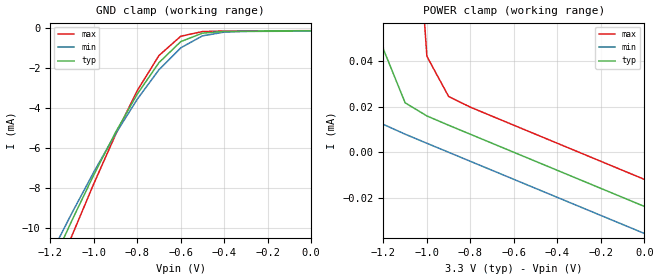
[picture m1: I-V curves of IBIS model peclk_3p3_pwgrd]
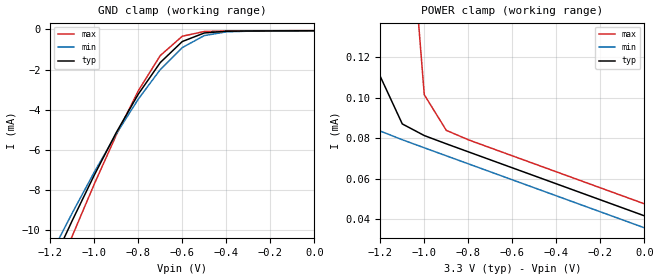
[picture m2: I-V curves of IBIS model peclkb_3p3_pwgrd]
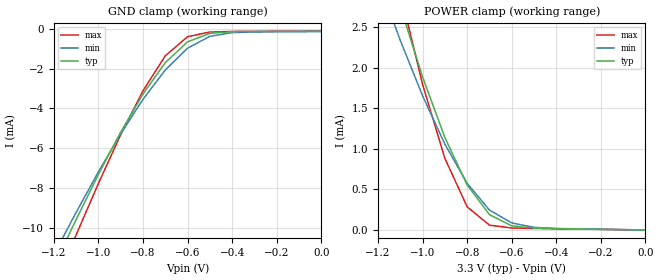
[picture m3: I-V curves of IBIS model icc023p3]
[IBIS ver]   2.1
[File name]   mpc9658.ibs
[File Rev]   2.2 {April 29, 2002}
[Date]   January 9th, 2002
[Disclaimer]   This information is for modeling purposes only
|   and is not guaranteed.
[Source]   Timing Solutions Operations
[Copyright]   Copyright 2001, Motorola Incorporated,
|   all rights reserved.
| Component MPC9658 for 3.3V Application!
[Component]   MPC96583p3
[Manufacturer]   Motorola
[Package]
|   typ   min   max
R_pkg   0.048   .038   0.053
L_pkg   6.045nH   5.084nH   7.950nH
C_pkg   0.813pF   0.560pF   1.157pF
[Pin]   signal_name model_name R_pin L_pin   C_pin
2   FB_IN   icc023p3   0.04   0.35nH   0.053pF
3   BYPASS_BAR  icc023p3   0.04   0.35nH   0.053pF
4   PLL_EN   icc023p3   0.04   0.35nH   0.053pF
5   MR/OEB   icc043p3   0.04   0.35nH   0.053pF
6   PCLK   peclk_3p3_pwgrd   0.04   0.35nH   0.053pF
7   PCLK_BAR   peclkb_3p3_pwgrd   0.04   0.35nH   0.053pF
10   Q9   occ013p3   0.04   0.35nH   0.053pF
12   Q8   occ013p3   0.04   0.35nH   0.053pF
14   Q7   occ013p3   0.04   0.35nH   0.053pF
16   Q6   occ013p3   0.04   0.35nH   0.053pF
18   Q5   occ013p3   0.04   0.35nH   0.053pF
20   Q4   occ013p3   0.04   0.35nH   0.053pF
22   Q3   occ013p3   0.04   0.35nH   0.053pF
24   Q2   occ013p3   0.04   0.35nH   0.053pF
26   Q1   occ013p3   0.04   0.35nH   0.053pF
28   Q0   occ013p3   0.04   0.35nH   0.053pF
30   QA1   occ013p3   0.04   0.35nH   0.053pF
32   VCO_SEL   icc023p3   0.04   0.35nH   0.053pF
|Component Inputs and Outputs at 2.5V Application
[Component]   MPC96582p5
[Manufacturer]   Motorola
[Package]
|   typ   min   max
R_pkg   0.048   .038   0.053
L_pkg   6.045nH   5.084nH   7.950nH
C_pkg   0.813pF   0.560pF   1.157pF
[Pin]   signal_name model_name R_pin L_pin   C_pin
2   FB_IN   icc022p5   0.04   0.35nH   0.053pF
3   BYPASS_BAR  icc022p5   0.04   0.35nH   0.053pF
4   PLL_EN   icc022p5   0.04   0.35nH   0.053pF
5   MR/OEB   icc042p5   0.04   0.35nH   0.053pF
6   PCLK   peclk_2p5_pwgrd   0.04   0.35nH   0.053pF
7   PCLK_BAR   peclkb_2p5_pwgrd   0.04   0.35nH   0.053pF
10   Q9   occ012p5   0.04   0.35nH   0.053pF
12   Q8   occ012p5   0.04   0.35nH   0.053pF
14   Q7   occ012p5   0.04   0.35nH   0.053pF
16   Q6   occ012p5   0.04   0.35nH   0.053pF
18   Q5   occ012p5   0.04   0.35nH   0.053pF
20   Q4   occ012p5   0.04   0.35nH   0.053pF
22   Q3   occ012p5   0.04   0.35nH   0.053pF
24   Q2   occ012p5   0.04   0.35nH   0.053pF
26   Q1   occ012p5   0.04   0.35nH   0.053pF
28   Q0   occ012p5   0.04   0.35nH   0.053pF
30   QA1   occ012p5   0.04   0.35nH   0.053pF
32   VCO_SEL   icc022p5   0.04   0.35nH   0.053pF
| Models and submodels in the file (10): peclk_3p3_pwgrd (Input), peclkb_3p3_pwgrd (Input), icc023p3 (Input), icc043p3 (Input), occ013p3 (Output), peclk_2p5_pwgrd (Input), peclkb_2p5_pwgrd (Input), icc042p5 (Input), icc022p5 (Input), occ012p5 (Output)
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|This is a Model of a PECL Input with a 25,000 ohm Pull_down at 3.3V
[Model]   peclk_3p3_pwgrd
Model_type   Input
Vmeas=1.5
Vinl=0.8
Vinh=2.0
| Variable   typ   min   max
C_comp   5p   5p   5p
[Temperature Range]   27.00   100.00   -45.00
[Power Clamp Reference]   3.30V   3.00V   3.60V
[Gnd Clamp Reference]   0.000V   0.000V   0.000V
[Voltage Range]   3.30V   3.00V   3.60V
[Pulldown Reference]   0.000V   0.000V   0.000V
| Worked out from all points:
|   GND clamp passes 1 mA (typ) near -0.63 V on its own axis
|   POWER clamp passes 1 mA (typ) near -1.46 V on its own axis
[GND_clamp]
| voltage   I(typ)   I(min)   I(max)
-3.3V     -65.58mA   -61.83mA   -70.36mA
-1.2V     -11.96mA   -11.35mA   -13.02mA
-1.1V     -9.594mA   -9.224mA   -10.36mA
-1V       -7.329mA   -7.188mA   -7.771mA
-900mV    -5.205mA   -5.279mA   -5.323mA
-800mV    -3.291mA   -3.546mA   -3.115mA
-700mV    -1.714mA   -2.069mA   -1.359mA
-600mV    -666.8uA   -975.9uA   -396.7uA
-500mV    -241.6uA   -377.6uA   -163.2uA
-400mV    -155.7uA   -192.2uA   -135.8uA
1.97fV    -130.7uA   -142.6uA   -118.8uA
[POWER_clamp]
| voltage   I(typ)  I(min)  I(max)
-3.3V     27.08mA    21.42mA    33.95mA
-1.5V     1.27mA     194.8uA    3.742mA
-1.4V     587.9uA    51.94uA    2.515mA
-1.3V     181.2uA    19.57uA    1.462mA
-1.2V     45.26uA    12.26uA    649.8uA
-1.1V     21.73uA    7.958uA    178.7uA
-1V       15.97uA    3.969uA    42.13uA
-900mV    11.89uA    5.703nA    24.5uA
-800mV    7.921uA    -3.955uA   19.82uA
1.97fV    -23.76uA   -35.64uA   -11.88uA
|This is a Model of a PECL_BAR Input with a 25,000 ohm Pull_Up at 3.3V
[Model]   peclkb_3p3_pwgrd
Model_type   Input
Vmeas=1.5
Vinl=.8
Vinh=2.0
| Variable   typ   min   max
C_comp   5p   5p   5p
[Temperature Range]   27.00   100.00   -45.00
[Power Clamp Reference]   3.30V   3.00V   3.60V
[Gnd Clamp Reference]   0.000V   0.000V   0.000V
[Voltage Range]   3.30V   3.00V   3.60V
[Pulldown Reference]   0.000V   0.000V   0.000V
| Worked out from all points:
|   GND clamp passes 1 mA (typ) near -0.64 V on its own axis
|   POWER clamp passes 1 mA (typ) near -1.45 V on its own axis
[GND_clamp]
| voltage   I(typ)   I(min)   I(max)
-3.3V     -65.51mA   -61.76mA   -70.3mA
-1.2V     -11.89mA   -11.28mA   -12.96mA
-1.1V     -9.53mA    -9.154mA   -10.3mA
-1V       -7.265mA   -7.118mA   -7.713mA
-900mV    -5.141mA   -5.209mA   -5.265mA
-800mV    -3.227mA   -3.475mA   -3.057mA
-700mV    -1.649mA   -1.999mA   -1.301mA
-600mV    -601.9uA   -905.3uA   -337.6uA
-500mV    -176.4uA   -306.5uA   -103.9uA
-400mV    -90.4uA    -121uA     -76.41uA
1.97fV    -65.34uA   -71.29uA   -59.4uA
[POWER_clamp]
| voltage   I(typ)  I(min)  I(max)
-3.3V     27.15mA    21.49mA    34.01mA
-1.5V     1.335mA    265.9uA    3.8mA
-1.4V     652.9uA    123.2uA    2.573mA
-1.3V     246.4uA    90.85uA    1.52mA
-1.2V     110.6uA    83.55uA    708.8uA
-1.1V     87.07uA    79.24uA    237.9uA
-1V       81.31uA    75.25uA    101.5uA
-900mV    77.23uA    71.29uA    83.9uA
-800mV    73.26uA    67.33uA    79.23uA
1.97fV    41.58uA    35.65uA    47.52uA
|This is a Model of an Input with a 25,000 ohm Pull_up at 3.3V
[Model]   icc023p3
Model_type   Input
Polarity   Non-Inverting
Vmeas=1.5
Vinl=0.8
Vinh=2.0
|Variable   typ   min   max
C_comp   5p   5p   5p
[Temperature Range]   27.00   100.00   -45.00
[Power Clamp Reference]   3.30V   3.00V   3.60V
[Gnd Clamp Reference]   0.000V   0.000V   0.000V
[Voltage Range]   3.30V   3.00V   3.60V
[Pulldown Reference]   0.000V   0.000V   0.000V
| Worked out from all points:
|   GND clamp passes 1 mA (typ) near -0.63 V on its own axis
|   POWER clamp passes 1 mA (typ) near -0.88 V on its own axis
[GND_clamp]
| voltage   I(typ)   I(min)   I(max)
-3.3V     -65.56mA   -61.83mA   -70.36mA
-1.2V     -11.94mA   -11.35mA   -13.02mA
-1.1V     -9.583mA   -9.224mA   -10.36mA
-1V       -7.318mA   -7.188mA   -7.771mA
-900mV    -5.193mA   -5.279mA   -5.323mA
-800mV    -3.28mA    -3.546mA   -3.115mA
-700mV    -1.702mA   -2.069mA   -1.359mA
-600mV    -655uA     -975.9uA   -396.7uA
-500mV    -229.7uA   -377.6uA   -163.2uA
-400mV    -143.9uA   -192.2uA   -135.8uA
1.97fV    -118.8uA   -142.6uA   -118.8uA
[POWER_clamp]
| voltage   I(typ)  I(min)  I(max)
-3.3V     32.89mA    26.85mA    40.63mA
-1.2V     3.727mA    3.095mA    4.229mA
-1.1V     2.756mA    2.338mA    2.93mA
-1V       1.886mA    1.654mA    1.795mA
-900mV    1.14mA     1.058mA    882.5uA
-800mV    554.8uA    575uA      285.5uA
-700mV    189.3uA    245.4uA    59.28uA
-600mV    51.31uA    86.95uA    24.32uA
-500mV    23.2uA     32.54uA    18.63uA
-400mV    16.45uA    18.02uA    14.85uA
0V        148.9pA    557.5pA    4.024pA
